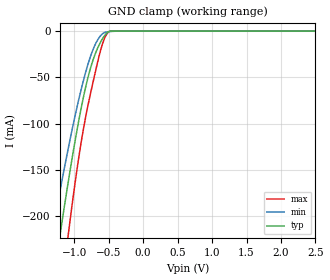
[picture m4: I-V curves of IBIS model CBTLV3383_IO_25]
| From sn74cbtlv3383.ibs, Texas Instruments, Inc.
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[Model]   CBTLV3383_IO_25
Model_type  Terminator
| variable   typ   min   max
C_comp   9.57pF   8.05pF   10.50pF
| C_tri-state   9.57pF   8.05pF   10.50pF
[Temperature Range]   40   100   -40
| Ambient temperature   25   85   -40
[Voltage range]   2.5   2.3   2.7
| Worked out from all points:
|   GND clamp passes 1 mA (typ) near -0.51 V on its own axis
[GND Clamp]
| CBTLV3383_IO_25
|   Voltage   I(typ)   I(min)   I(max)
-2.5V     -974.5mA   -778.2mA   -1.258A
-1.315V   -276.4mA   -217.4mA   -365.5mA
-1.205V   -220.2mA   -172.5mA   -293.4mA
-1.18V    -207.8mA   -162.6mA   -277.6mA
-1.09V    -164.6mA   -128.1mA   -222.3mA
-1.07V    -155.4mA   -120.7mA   -210.5mA
-945mV    -101.2mA   -77.46mA   -142.2mA
-815mV    -54.54mA   -39.5mA    -85.68mA
-695mV    -24.66mA   -14.45mA   -44.69mA
-570mV    -5.963mA   -1.922mA   -9.721mA
-475mV    -100.2uA   -453.8uA   -60.55uA
2.5V      1.375nA    62.46nA    18.69pA
